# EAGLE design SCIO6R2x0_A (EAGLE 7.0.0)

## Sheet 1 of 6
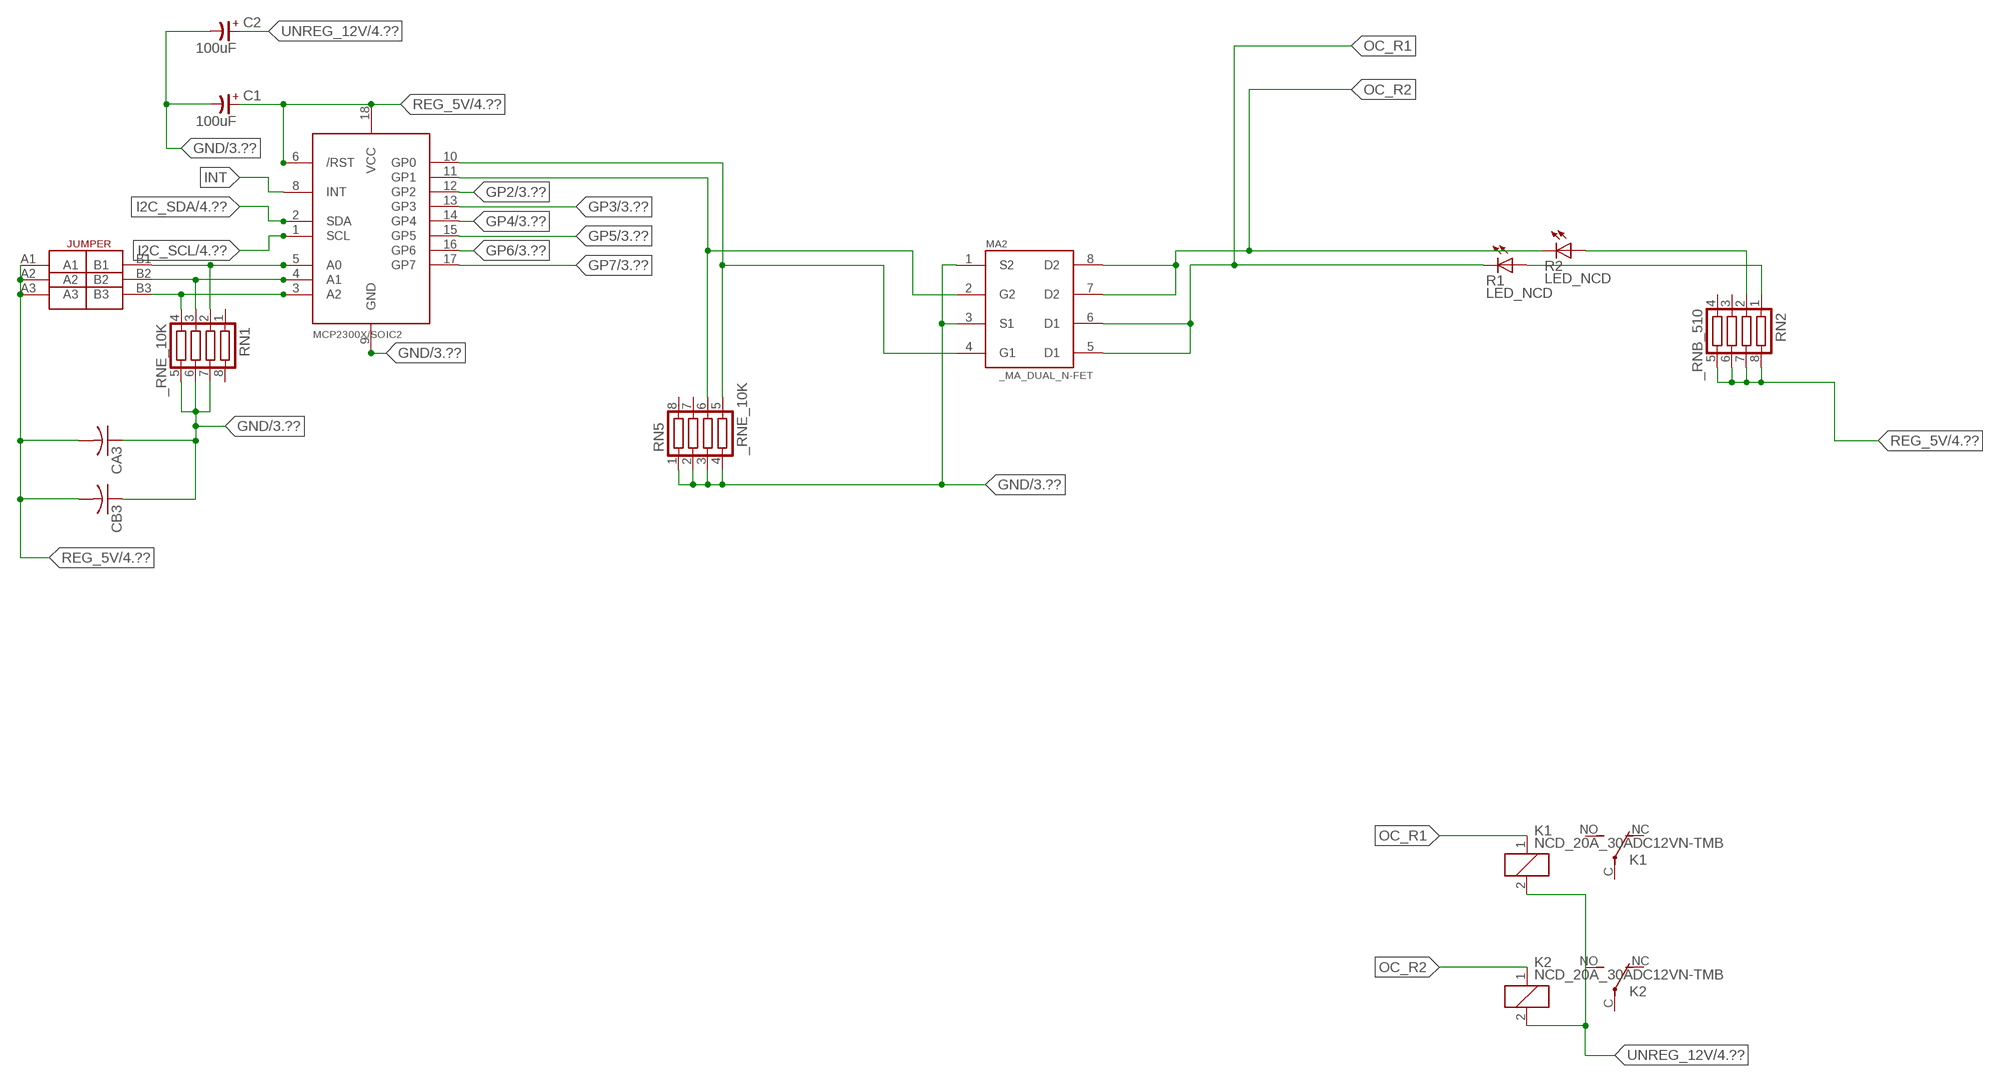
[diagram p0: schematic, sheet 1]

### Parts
C1  100uF  CP-E-025X060  [E-025X060]
C2  100uF  CP-E-025X060  [E-025X060]
CA3  CC1206KRX7R9BB104C1206K  [CC1206KRX7R9BB104]
CB3  TMK316F106ZL-TC1206K  [TMK316F106ZL-T]
IC2  MCP2300X/SO  [SO18W]
K1  NCD_20A_30ADC12VN-TMB  [JT-TMB]
K2  NCD_20A_30ADC12VN-TMB  [JT-TMB]
MA2  _MA_DUAL_N-FET  [_MA_DUAL_N-FET]
R1  LED_NCD  [CHIPLED_0603]
R2  LED_NCD  [CHIPLED_0603]
RN1  _RNE_10K  [RNE]
RN2  _RNB_510  [RNB]
RN5  _RNE_10K  [RNE]
U$18  JUMPER_3X2  [JUMPER_3X2]

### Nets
GND: C1.- C2.- CA3.1 CB3.1 IC2.9(GND) MA2.1(S2) MA2.3(S1) RN1.5 RN1.6 RN1.7 RN5.1 RN5.2 RN5.3 RN5.4 ; also sheet 3,4,6
GP2: IC2.12(GP2) ; also sheet 3
GP3: IC2.13(GP3) ; also sheet 3
GP4: IC2.14(GP4) ; also sheet 3
GP5: IC2.15(GP5) ; also sheet 3
GP6: IC2.16(GP6) ; also sheet 3
GP7: IC2.17(GP7) ; also sheet 3
I2C_SCL: IC2.1(SCL) ; also sheet 4
I2C_SDA: IC2.2(SDA) ; also sheet 4
INT: IC2.8(INT)
N$6: IC2.5(A0) RN1.2 U$18.B1
N$7: IC2.4(A1) RN1.3 U$18.B2
N$8: IC2.3(A2) RN1.4 U$18.B3
N$22: IC2.11(GP1) MA2.2(G2) RN5.6
N$23: IC2.10(GP0) MA2.4(G1) RN5.5
N$31: R2.A RN2.2
N$32: R1.A RN2.1
OC_R1: K1.1(C1) MA2.5(D1) MA2.6(D1) R1.C
OC_R2: K2.1(C1) MA2.7(D2) MA2.8(D2) R2.C
REG_5V: C1.+ CA3.2 CB3.2 IC2.6(/RST) IC2.18(VCC) RN2.5 RN2.6 RN2.7 RN2.8 U$18.A1 U$18.A2 U$18.A3 ; also sheet 4,6
UNREG_12V: C2.+ K1.2(C2) K2.2(C2) ; also sheet 4
Unconnected: K1.C(COM) K1.NC K1.NO K2.C(COM) K2.NC K2.NO RN1.1 RN1.8 RN2.3 RN2.4 RN5.7 RN5.8

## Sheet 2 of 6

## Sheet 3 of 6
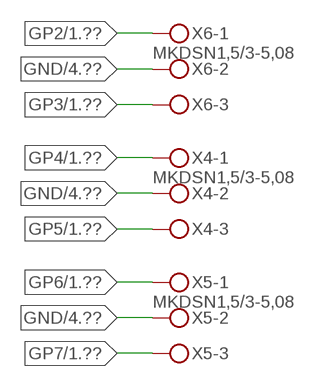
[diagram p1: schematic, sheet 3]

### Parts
X4  MKDSN1,5/3-5,08  [MKDSN1,5/3-5,08]
X5  MKDSN1,5/3-5,08  [MKDSN1,5/3-5,08]
X6  MKDSN1,5/3-5,08  [MKDSN1,5/3-5,08]

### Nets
GND: X4.2 X5.2 X6.2 ; also sheet 1,4,6
GP2: X6.1 ; also sheet 1
GP3: X6.3 ; also sheet 1
GP4: X4.1 ; also sheet 1
GP5: X4.3 ; also sheet 1
GP6: X5.1 ; also sheet 1
GP7: X5.3 ; also sheet 1

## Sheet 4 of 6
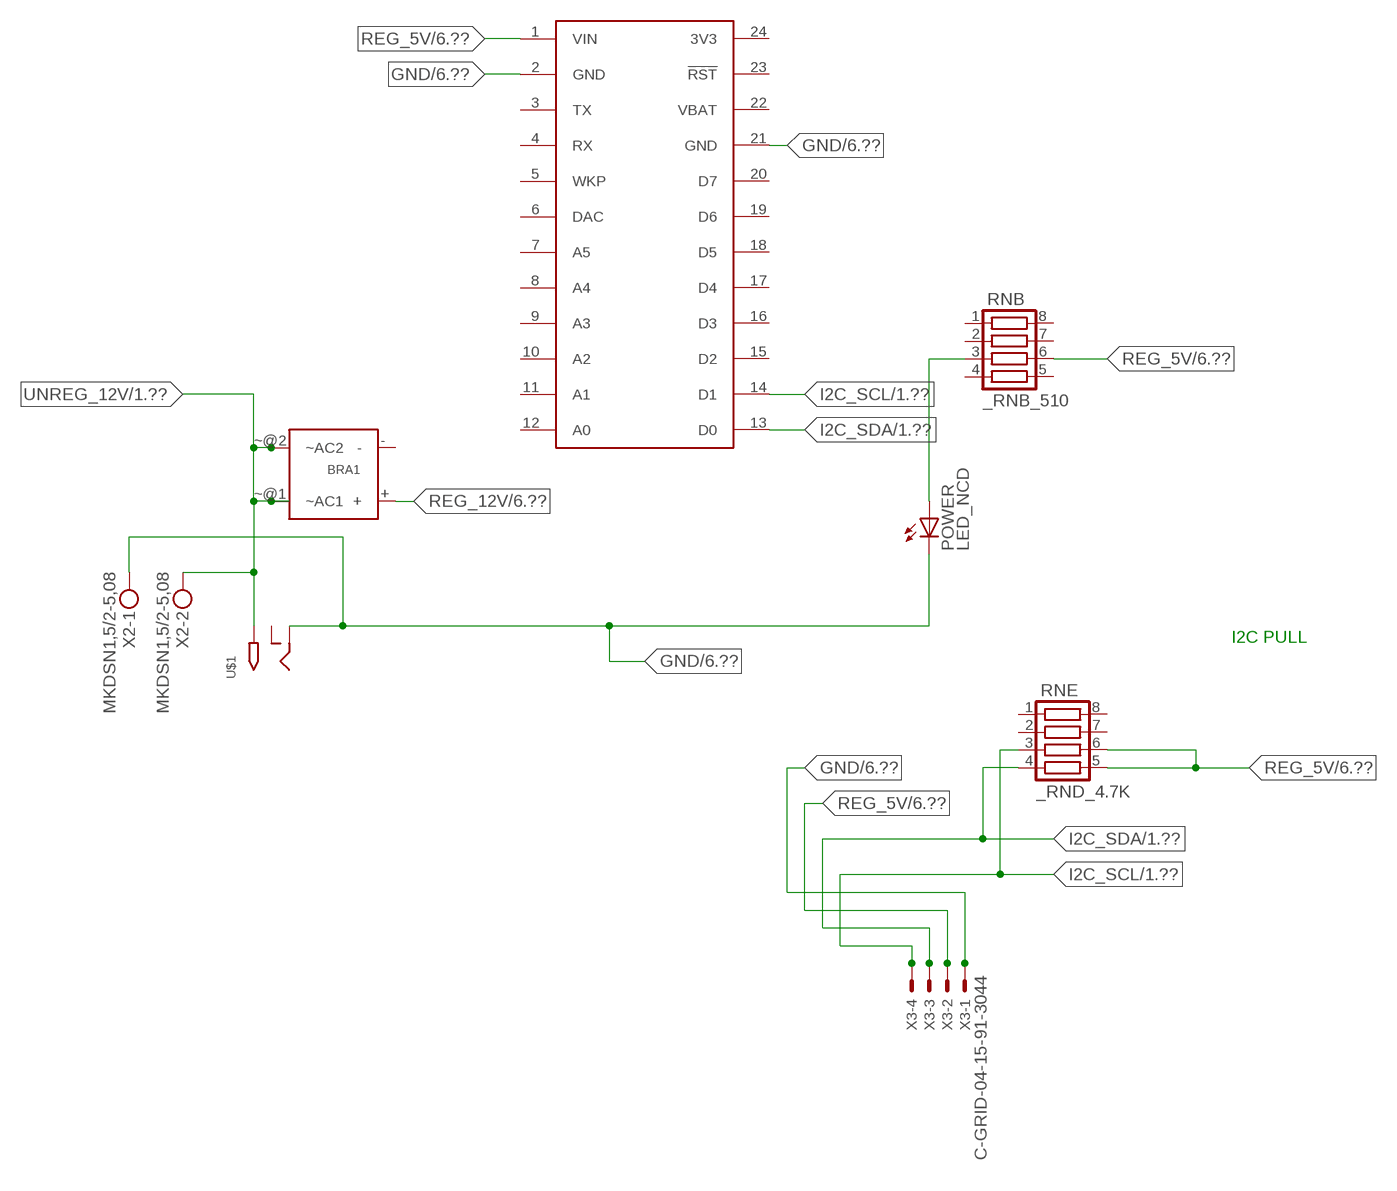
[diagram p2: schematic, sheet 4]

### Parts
BRA1  MB2S_  [MB2S]
POWER  LED_NCD  [CHIPLED_0603]
RNB  _RNB_510  [RNB]
RNE  _RND_4.7K  [RND]
S1  SPARK_CORECORE  [SPARK_CORE]
U$1  2.1MMJACK  [PJ-102A]
X2  MKDSN1,5/2-5,08  [MKDSN1,5/2-5,08]
X3  C-GRID-04-15-91-3044  [15-91-04]

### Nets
GND: POWER.C S1.2(GND) S1.21(GND) U$1.RING X2.1 X3.1 ; also sheet 1,3,6
I2C_SCL: RNE.3 S1.14(D1) X3.4 ; also sheet 1
I2C_SDA: RNE.4 S1.13(D0) X3.3 ; also sheet 1
N$2: POWER.A RNB.3
REG_5V: RNB.6 RNE.5 RNE.6 S1.1(VIN) X3.2 ; also sheet 1,6
REG_12V: BRA1.+ ; also sheet 6
UNREG_12V: BRA1.~@1(~AC1) BRA1.~@2(~AC2) U$1.TIP X2.2 ; also sheet 1
Unconnected: BRA1.- RNB.1 RNB.2 RNB.4 RNB.5 RNB.7 RNB.8 RNE.1 RNE.2 RNE.7 RNE.8 S1.3(TX) S1.4(RX) S1.5(WKP) S1.6(DAC) S1.7(A5) S1.8(A4) S1.9(A3) S1.10(A2) S1.11(A1) S1.12(A0) S1.15(D2) S1.16(D3) S1.17(D4) S1.18(D5) S1.19(D6) S1.20(D7) S1.23(!RST) U$1.RING_SW

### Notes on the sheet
- I2C PULL

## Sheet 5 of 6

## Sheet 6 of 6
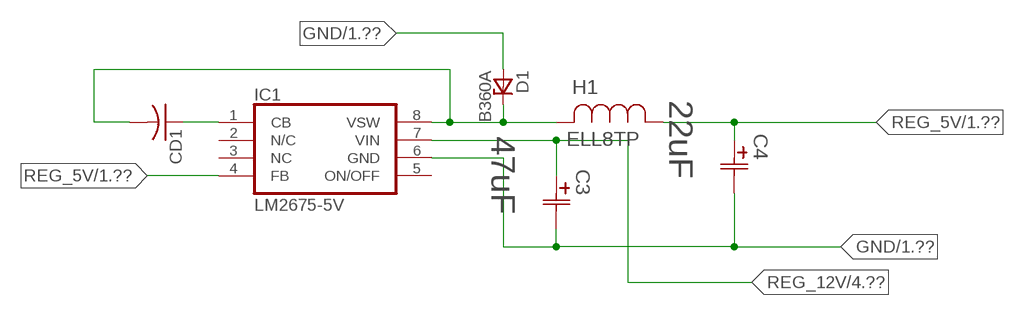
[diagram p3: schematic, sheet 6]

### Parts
C3  47uF  490-5463-6-NDCAP  [C2917(7343)-Y]
C4  22uF  490-5463-6-NDCAP  [C2917(7343)-Y]
CD1  _CD_10NF_50VC1206K  [_CD_10NF_50V]
D1  B360A  [DO214AC_ZENER]
H1  ELL8TP  [IND_ELL8TP]
IC1  LM2675-5V  LM2675  [SO-8]

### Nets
GND: C3.2(C2) C4.2(C2) D1.A IC1.6(GND) ; also sheet 1,3,4
N$1: CD1.2 D1.C H1.2 IC1.8(VSW)
N$3: CD1.1 IC1.1(CB)
REG_5V: C4.1(C1) H1.1 IC1.4(FB) ; also sheet 1,4
REG_12V: C3.1(C1) IC1.7(VIN) ; also sheet 4
Unconnected: IC1.2(N/C) IC1.5(ON/OFF)

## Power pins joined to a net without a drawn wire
3V3: S1.24(3V3)
NC: IC1.3(NC)
VBAT: S1.22(VBAT)

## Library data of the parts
BRA1 = NCD_ULTIMATE_LIBRARY:MB2S: Bridge Rectifier BRA MB2S 200V 500ma Digikey MB2S-TPMSTR-ND/MB2S-TP
C1 C2 = NCD_ULTIMATE_LIBRARY:CP-: Capacitors All Kinds POLARIZED CAP
C3 C4 = NCD_ULTIMATE_bhaskar:490-5463-6-ND: NCD CAP
CA3 = NCD_ULTIMATE_LIBRARY:CC1206KRX7R9BB104: Capacitor CA .1uF 50V SMT C1206K CC1206KRX7R9BB104
CB3 = NCD_ULTIMATE_LIBRARY:TMK316F106ZL-T: Capacitor CB 10uF SMT 1206 TMK316F106ZL-T
CD1 = NCD_ULTIMATE_LIBRARY:_CD_10NF_50V: Capacitor 10nF SMT
D1 = NCD_ULTIMATE_bhaskar:B360A: NCD DIODE B350A/B360A
H1 = NCD_ULTIMATE_bhaskar:ELL8TP: NCD coil
IC1 = NCD_ULTIMATE_bhaskar:LM2675: LM2675 NCD http://www.ti.com/lit/ds/symlink/lm2675.pdf
IC2 = NCD_ULTIMATE_LIBRARY:MCP2300X: Semiconductor Port Expander I/O 8-Bit I2C MCP23008 Inexpensive i2c i/o expander - 8 general purpose i/o pins with optional pullups
K1 K2 = NCD_ULTIMATE_LIBRARY:NCD_20A_30A: RELAY COMPACT ECONOMICAL 30 AMP. RELAY NAiS Source: http://www.mew-europe.com/.. en_ds_61212_0000.pdf
MA2 = NCD_ULTIMATE_LIBRARY:_MA_DUAL_N-FET: FET Dual N-Channel 8-SOIC NMOSFET Digikey 785-1064-2-ND/AO4842
POWER = NCD_ULTIMATE_bhaskar:LED_NCD
R1 R2 = NCD_ULTIMATE_LIBRARY:LED_NCD: LED Digikey 754-1132-2-ND/APT2012SRCPRV
RN1 RN5 = NCD_ULTIMATE_LIBRARY:_RNE_10K: Resistor Array RNE SMT 10K x 4 Single Resistor Source: http://www.ctscorp.com/components/Datasheets/CTSChipArrayDs.pdf Digikey 742C083103JPTR-ND/742C083103JP; OC_FARNELL: unknown; OC_NEWARK: unknown
RN2 RNB = NCD_ULTIMATE_LIBRARY:_RNB_510: Resistor Array RNB SMT 510 x 4 Single Resistor Source: http://www.ctscorp.com/components/Datasheets/CTSChipArrayDs.pdf Digikey 742C083511JPTR-ND/ 742C083511JP; OC_FARNELL: unknown; OC_NEWARK: unknown
RNE = NCD_ULTIMATE_LIBRARY:_RND_4.7K: Resistor Array RND SMT 4.7K x 4 Single Resistor Source: http://www.ctscorp.com/components/Datasheets/CTSChipArrayDs.pdf Digikey 742C083472JPTR-ND/742C083472JP; OC_FARNELL: unknown; OC_NEWARK: unknown
S1 = Spark:SPARK_CORE
U$1 = NCD_ULTIMATE_CONNECTORS:2.1MMJACK: 2.1mm x 5.5mm DC jack with internal switch. Digikey part #PJ-102A, 4UCON part #05537 By microbuilder.eu
U$18 = NCD_ULTIMATE_CONNECTORS:JUMPER_3X2
X2 = NCD_ULTIMATE_CONNECTORS:MKDSN1,5/2-5,08: MKDSN 1,5/ 2-5,08 Printklemme
X3 = NCD_ULTIMATE_CONNECTORS:C-GRID-04: CONNECTOR 4-Pos I2C wire to board 2.54 mm (0.100") pitch header Digikey WM1342-ND/0015912045; OC_FARNELL: unknown; OC_NEWARK: unknown
X4-X6 = NCD_ULTIMATE_CONNECTORS:MKDSN1,5/3-5,08: MKDSN 1,5/ 3-5,08 Printklemme Nennstrom: 13,5 A Nennspannung: 250 V Rastermaß: 5,08 mm Polzahl: 3 Anschlussart: Schraubanschluss Montage: Löten Anschlussrichtung Leiter/Platine: 0 ° Artikelnummer: 1729131 Source: http://eshop.phoenixcontact.com .. 1729131.pdf

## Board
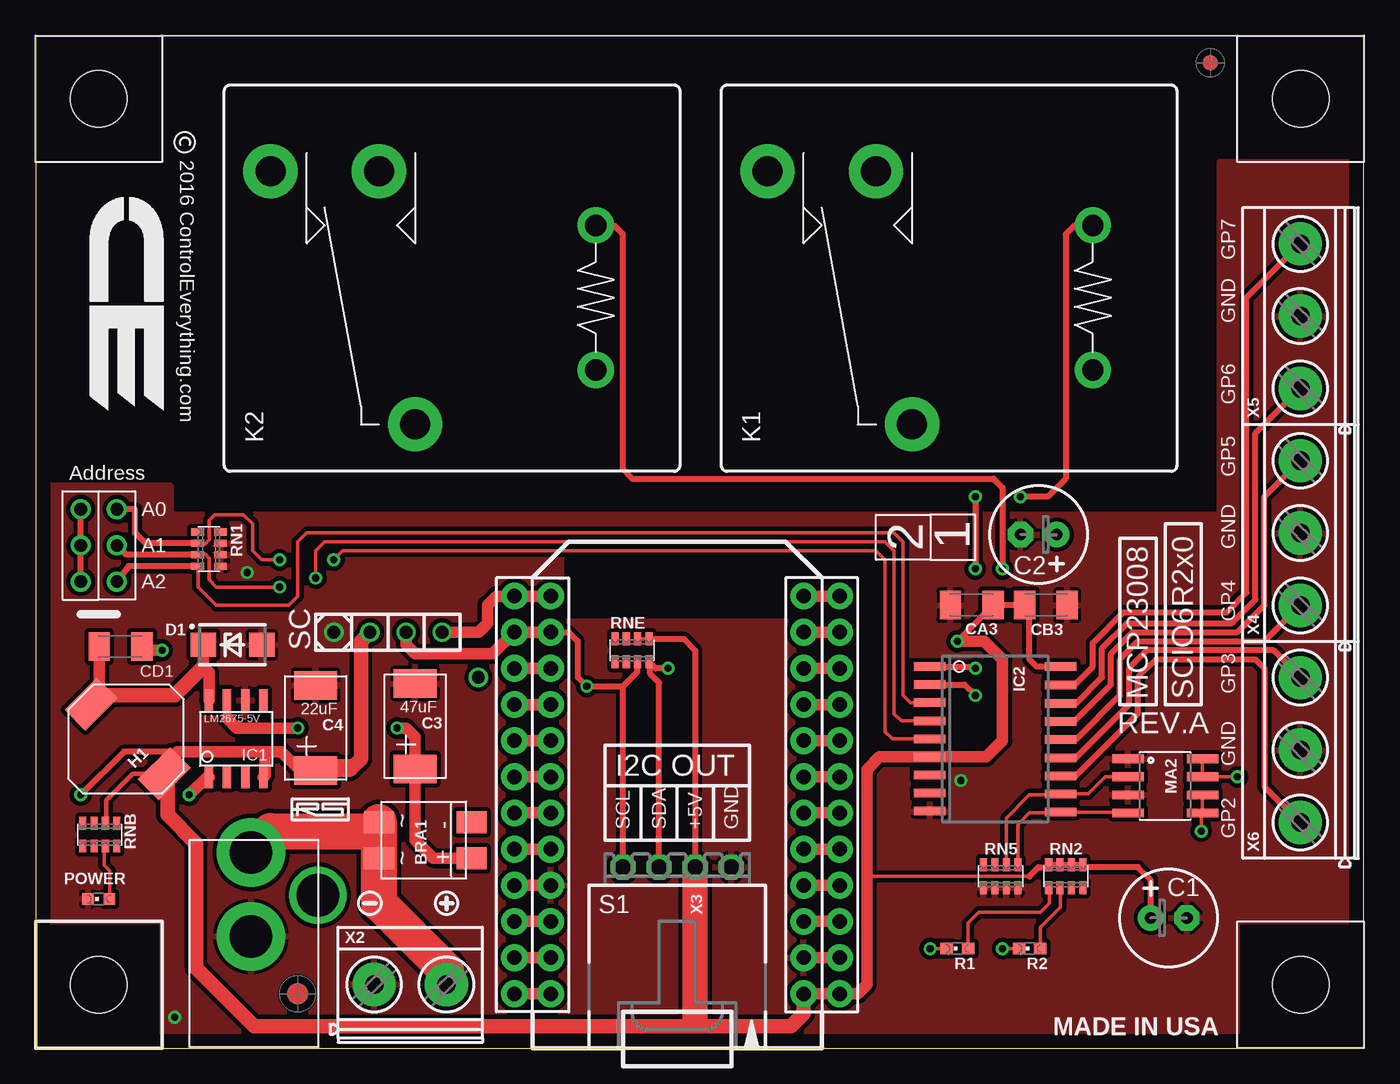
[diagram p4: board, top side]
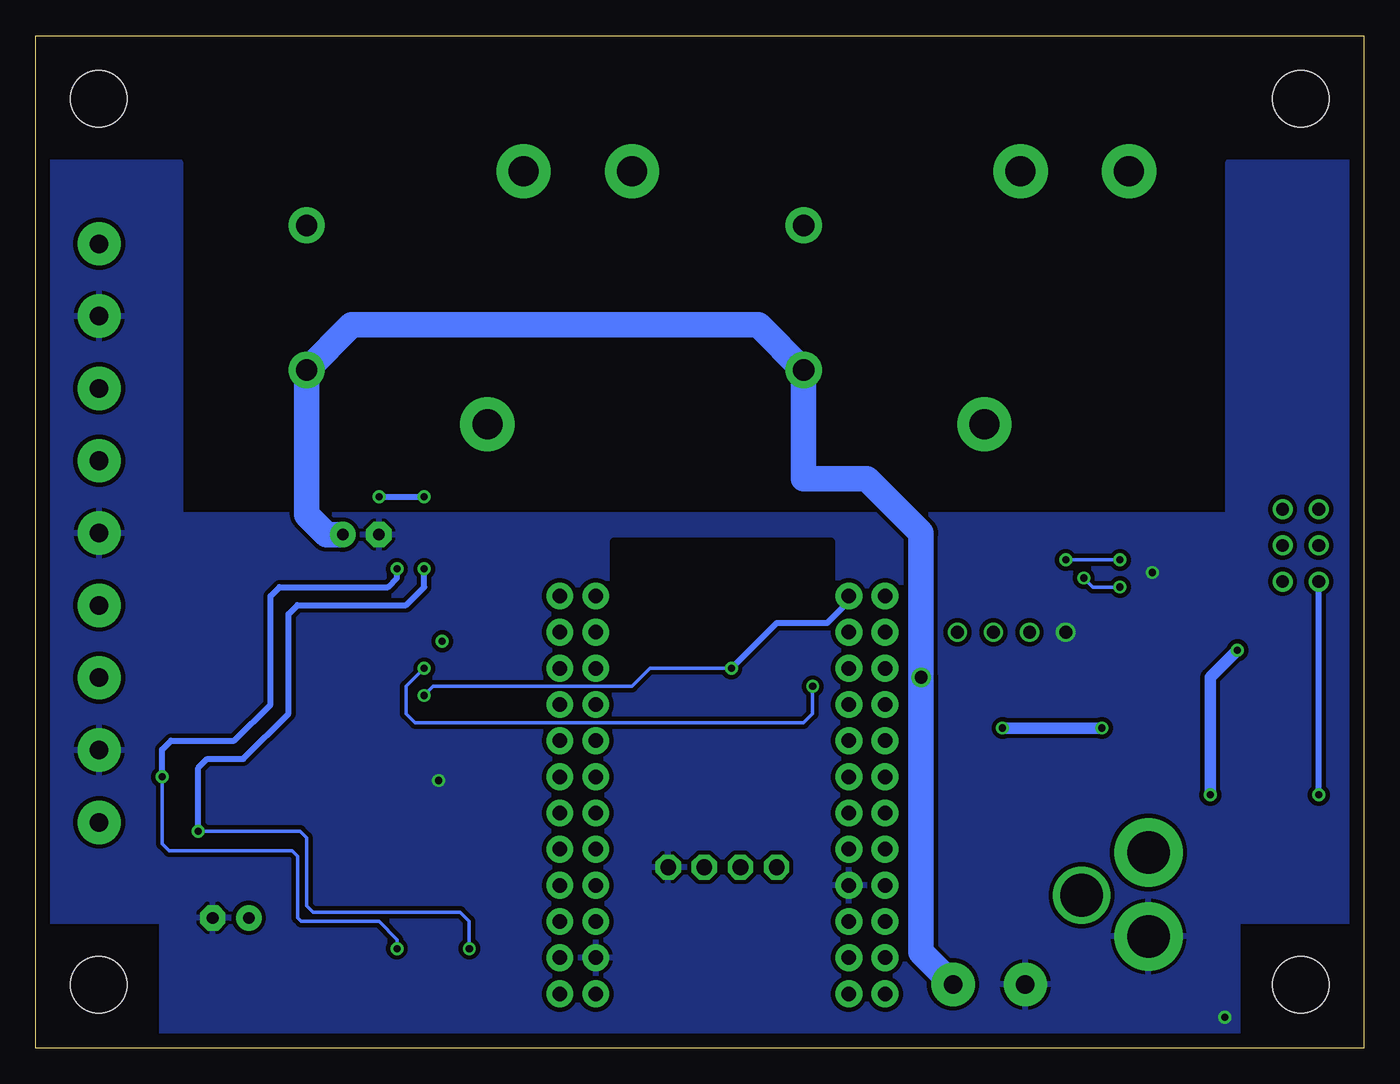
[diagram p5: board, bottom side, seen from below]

Size 93.34 x 71.12 mm. Coordinates in mm from the lower left corner, seen from the top.
Outline: 0,59.99 0,59.05
Outline: 0,59.05 0,0 75.56,0 93.34,0 93.34,71.12 0,71.12 0,59.05
Copper layers (1*16): Top 0.035mm / dielectric 1.5mm / Bottom 0.035mm
Design rules "default": minimum track width 10mil, minimum drill 24mil, track to track 8mil, track to pad 8mil, pad to pad 8mil, via to via 8mil, smd to smd 8mil, copper to edge 40mil, drill to drill 8mil, minimum pad ring 10mil, minimum via ring 8mil, stop-mask expansion 4mil, vias tented up to drill 0mil, thermal gap 10mil
Holes 3.96 mm at 4.45,4.45 4.45,4.45

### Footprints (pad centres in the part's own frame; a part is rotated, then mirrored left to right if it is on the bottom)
MB2S = smd 1.55 x 2.1: + 0,-6.5; - 2.54,-6.5; ~@1 0,0; ~@2 2.54,0
E-025X060 = drill 0.813 pad 1.778: + -1.27,0 | drill 0.813 pad 1.778 octagon: - 1.27,0
C2917(7343)-Y = smd 2 x 3: 1 -3,0; 2 3,0
CC1206KRX7R9BB104 = smd 1.5 x 2: 1 -1.5,0; 2 1.5,0
TMK316F106ZL-T = smd 1.5 x 2: 1 -1.5,0; 2 1.5,0
_CD_10NF_50V = smd 1.5 x 2: 1 -1.5,0; 2 1.5,0
DO214AC_ZENER = smd 1.8 x 1.7: A 2.05,0; C -2.05,0
IND_ELL8TP = smd 2.054 x 3.2 rotated 45: 1 -2.442,-2.696; 2 2.442,2.442
SO-8 = smd 0.6 x 1.55: 1 -1.905,-2.69; 2 -0.635,-2.69; 3 0.635,-2.69; 4 1.905,-2.69; 5 1.905,2.71; 6 0.635,2.71; 7 -0.635,2.71; 8 -1.905,2.71
SO18W = smd 0.6 x 2.2: 1 -4.445,-4.6; 2 -3.175,-4.6; 3 -1.905,-4.6; 4 -0.635,-4.6; 5 0.635,-4.6; 6 1.905,-4.6; 7 3.175,-4.6; 8 4.445,-4.6; 9 5.715,-4.6; 10 5.775,4.6; 11 4.505,4.6; 12 3.235,4.6; 13 1.965,4.6; 14 0.695,4.6; 15 -0.575,4.6; 16 -1.845,4.6; 17 -3.145,4.6; 18 -4.445,4.6
JT-TMB = drill 1.5 pad 2.54: 1 5.08,0; 2 -5.08,0 | drill 2.1 pad 3.81: C -8.89,12.7; NC 8.89,22.86; NO 8.89,15.24
_MA_DUAL_N-FET = smd 0.61 x 2.21: 1 -1.905,-2.616; 2 -0.635,-2.616; 3 0.635,-2.616; 4 1.905,-2.616; 5 1.905,2.616; 6 0.635,2.616; 7 -0.635,2.616; 8 -1.905,2.616
CHIPLED_0603 = smd 0.8 x 0.8: A 0,-0.75; C 0,0.75
CHIPLED_0603' = smd 0.8 x 0.876: A 0,-0.75; C 0,0.75
RNE = smd 0.5 x 0.9: 1 -1.2,-0.8; 2 -0.4,-0.8; 3 0.4,-0.8; 4 1.2,-0.8; 5 1.2,0.8; 6 0.4,0.8; 7 -0.4,0.8; 8 -1.2,0.8
RNB = smd 0.5 x 0.9: 1 -1.2,-0.8; 2 -0.4,-0.8; 3 0.4,-0.8; 4 1.2,-0.8; 5 1.2,0.8; 6 0.4,0.8; 7 -0.4,0.8; 8 -1.2,0.8
RND = smd 0.5 x 0.9: 1 -1.2,-0.8; 2 -0.4,-0.8; 3 0.4,-0.8; 4 1.2,-0.8; 5 1.2,0.8; 6 0.4,0.8; 7 -0.4,0.8; 8 -1.2,0.8
SPARK_CORE = drill 1.016 pad 1.88: 1 -8.89,13.97; 2 -8.89,11.43; 3 -8.89,8.89; 4 -8.89,6.35; 5 -8.89,3.81; 6 -8.89,1.27; 7 -8.89,-1.27; 8 -8.89,-3.81; 9 -8.89,-6.35; 10 -8.89,-8.89; 11 -8.89,-11.43; 12 -8.89,-13.97; 13 8.89,-13.97; 14 8.89,-11.43; 15 8.89,-8.89; 16 8.89,-6.35; 17 8.89,-3.81; 18 8.89,-1.27; 19 8.89,1.27; 20 8.89,3.81; 21 8.89,6.35; 22 8.89,8.89; 23 8.89,11.43; 24 8.89,13.97; 25 -11.43,13.97; 26 -11.43,11.43; 27 -11.43,8.89; 28 -11.43,6.35; 29 -11.43,3.81; 30 -11.43,1.27; 31 -11.43,-1.27; 32 -11.43,-3.81; 33 -11.43,-6.35; 34 -11.43,-8.89; 35 -11.43,-11.43; 36 -11.43,-13.97; 37 11.43,13.97; 38 11.43,11.43; 39 11.43,8.89; 40 11.43,6.35; 41 11.43,3.81; 42 11.43,1.27; 43 11.43,-1.27; 44 11.43,-3.81; 45 11.43,-6.35; 46 11.43,-8.89; 47 11.43,-11.43; 48 11.43,-13.97
PJ-102A = drill 3 pad 4.8: RING 0.1,-3.39; TIP 0.1,-9.29 | drill 3 pad 3.251: RING_SW -4.6,-6.29
PCB_MOUNTING_HOLE = hole 3.962: 4.445,4.445
JUMPER_3X2 = drill 0.9: A1 0,5.08; A2 0,2.54; A3 0,0; B1 2.54,5.08; B2 2.54,2.54; B3 2.54,0
MKDSN1,5/2-5,08 = drill 1.3 pad 3.048: 1 -2.561,0.025; 2 2.519,0.025
15-91-04 = drill 1.1 pad 1.778 octagon: 1 -3.81,-7.62; 2 -1.27,-7.62; 3 1.27,-7.62; 4 3.81,-7.62
MKDSN1,5/3-5,08 = drill 1.3 pad 3.048: 1 -7.641,0.025; 2 -2.561,0.025; 3 2.519,0.025

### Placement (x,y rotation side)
BRA1  24.13,13.34 90 top
C1  79.63,9.14 0 top
C2  70.48,36.07 180 top
C3  26.67,22.61 90 top
C4  19.68,22.48 90 top
CA3  65.79,31.12 0 top
CB3  70.99,31.12 180 top
CD1  5.97,28.19 180 top
D1  13.84,28.32 0 top
H1  6.35,21.72 90 top
IC1  14.1,21.72 0 top
IC2  67.44,22.35 270 top
K1  74.3,52.7 90 top
K2  39.37,52.7 90 top
MA2  79.38,18.41 270 top
POWER  4.45,10.48 90 top
R1  LED_NCD  [CHIPLED_0603']  64.77,6.98 90 top
R2  LED_NCD  [CHIPLED_0603']  69.85,6.98 90 top
RN1  12.19,35.05 270 top
RN2  72.39,12.07 0 top
RN5  67.82,12.07 0 top
RNB  4.51,14.99 0 top
RNE  41.91,27.94 0 top
S1  45.09,17.78 180 top
U$1  15.24,4.45 180 top
U$4  PCB_MOUNTING_HOLE  [PCB_MOUNTING_HOLE]  93.34,62.23 90 top
U$6  PCB_MOUNTING_HOLE  [PCB_MOUNTING_HOLE]  93.34,0 90 top
U$10  [VISION_REF15]  18.41,3.81 0 top
U$11  PCB_MOUNTING_HOLE  [PCB_MOUNTING_HOLE]  8.89,62.23 90 top
U$18  3.17,32.77 0 top
U$19  [VISION_REF10]  82.55,69.22 0 top
U$21  [ICON_USA]  71.5,0.89 0 top
U$22  [ICON_MINUS]  23.5,10.16 180 top
U$24  [ICON_PLUS]  28.89,10.16 90 top
X2  26.35,4.45 0 top
X3  45.09,5.08 180 top
X4  88.9,38.73 90 top
X5  88.9,53.97 90 top
X6  88.9,23.5 90 top

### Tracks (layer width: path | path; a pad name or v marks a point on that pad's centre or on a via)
GND  (via drill 0.5, 0.9)
  other vias: 14.86,33.4 65.02,18.8 9.78,2.16 20.95,29.21
  pour Bottom (isolate 0.305): -1.91,8.89 8.89,8.89 8.89,0 84.45,0 84.45,8.89 92.71,8.89 92.71,62.23 83.19,62.23 83.19,37.46 9.53,37.46 9.53,62.23 -1.91,62.23
  pour Top (isolate 0.305): -3.81,8.89 8.89,8.89 8.89,0 84.45,0 84.45,8.89 92.71,8.89 92.71,62.23 83.19,62.23 83.19,37.46 9.53,37.46 9.53,39.5 -3.81,39.5
GP2
  Top 0.406: IC2.12 73.09,19.12 77.47,23.5 77.47,26.04 78.74,27.3 85.72,27.3 86.36,26.67 86.36,18.37 X6.1
GP3
  Top 0.406: X6.3 88.88,26.06 87,27.94 78.11,27.94 76.83,26.67 76.83,24.13 73.03,20.32 72.1,20.32 IC2.13
GP4
  Top 0.406: IC2.14 73.09,21.66 76.2,24.77 76.2,27.3 77.47,28.57 86.36,28.57 X4.1
GP5
  Top 0.406: IC2.15 72.97,22.93 75.56,25.53 75.56,27.69 77.09,29.21 84.45,29.21 86.36,31.12 86.36,38.74 X4.3
GP6
  Top 0.406: IC2.16 73.09,24.2 74.93,26.04 74.93,28.07 76.71,29.85 84.07,29.85 85.72,31.5 85.72,43.18 X5.1
GP7
  Top 0.406: IC2.17 73,25.5 74.3,26.8 74.3,28.45 76.45,30.61 83.69,30.61 85.09,32 85.09,52.71 X5.3
I2C_SCL  (via drill 0.5, 0.9)
  Top 0.406: IC2.1 65.91,26.8 v66.04,26.67 | X3.4 41.27,25.4 | 41.27,25.4 42.29,26.42 42.29,27.12 RNE.3 | S1.14 37.47,29.21 38.1,28.57 38.1,26.04 v38.73,25.4 41.27,25.4
  Top 0.813: v26.04,29.21 26.04,28.32 26.67,27.69 32.13,27.69 33.66,29.21
  Bottom 0.254: v38.73,25.4 38.73,23.5 39.37,22.86 66.67,22.86 67.31,23.5 67.31,25.4 v66.04,26.67
I2C_SDA  (via drill 0.5, 0.9)
  Top 0.406: IC2.2 65.28,25.53 v66.04,24.77 | X3.3 43.81,25.65 43.18,26.29 43.18,27.07 RNE.4 43.58,26.67 v44.45,26.67
  Top 0.813: v28.57,29.21 31.11,29.21 31.75,29.85 31.75,31.12 32.38,31.75 33.66,31.75
  Bottom 0.254: v44.45,26.67 50.16,26.67 51.44,25.4 65.41,25.4 v66.04,24.77
  Bottom 0.406: S1.13 36.2,31.37 37.72,29.85 41.27,29.85 v44.45,26.67
N$1
  Top 0.813: H1.2 3.88,24.77 | D1.C 11.79,26.78 12.19,26.38 IC1.8 | CD1.2 4.47,24.79 4.45,24.77
  Top 1.016: 3.88,24.77 4.45,24.77 9.78,24.77 11.79,26.78
N$2
  Top 0.254: POWER.A 5.2,12.46 4.83,12.83 4.83,14.1 RNB.3
  Top 0.406: 4.95,14.14 RNB.3
N$3  (via drill 0.5)
  Top 0.813: IC1.1 12.04,19.03 v10.79,17.78 | v8.89,27.94 7.72,27.94 CD1.1
  Bottom 0.813: v10.79,17.78 10.79,26.04 v8.89,27.94
N$6  (via drill 0.5)
  Top 0.254: IC2.5 60.2,21.72 59.69,22.23 59.69,34.29 59.05,34.92 21.59,34.92 v20.95,34.29 | v17.14,34.29 15.88,34.29 15.24,34.92 15.24,36.83 14.61,37.46 12.57,37.46 12.19,37.08 12.19,35.69 11.94,35.43 11.41,35.43 RN1.2
  Top 0.406: RN1.2 7.73,35.45 6.99,36.2 6.99,37.85 U$18.B1
  Bottom 0.254: v20.95,34.29 v17.14,34.29
N$7  (via drill 0.5)
  Top 0.254: IC2.4 60.83,22.99 60.33,23.5 60.33,34.92 59.69,35.56 20.32,35.56 19.68,34.92 v19.68,33.02 | v17.14,32.38 12.7,32.38 12.19,32.89 12.19,34.42 11.94,34.67 11.41,34.67 RN1.3
  Top 0.406: RN1.3 6.37,34.65 U$18.B2
  Bottom 0.254: v19.68,33.02 19.05,32.38 v17.14,32.38
N$8
  Top 0.254: IC2.3 61.47,24.26 60.96,24.77 60.96,35.56 60.33,36.2 19.05,36.2 18.41,35.56 18.41,31.75 17.78,31.12 12.7,31.12 11.43,32.38 11.43,33.81 RN1.4
  Top 0.406: RN1.4 6.53,33.85 U$18.B3
N$22
  Top 0.254: MA2.2 75.18,19.05 73.98,17.85 IC2.11 71.97,17.78 69.85,17.78 68.22,16.15 RN5.6
N$23
  Top 0.254: MA2.4 76.69,16.58 IC2.10 71.97,16.51 69.85,16.51 69.02,15.68 RN5.5
N$31
  Top 0.254: R2.A 70.6,8.5 72.01,9.91 72.01,11.25 RN2.2
N$32
  Top 0.254: R1.A 65.52,8.75 66.29,9.52 70.61,9.52 71.25,10.16 71.25,11.21 RN2.1
OC_R1  (via drill 0.5)
  Top 0.254: R1.C v62.87,6.98 | v81.92,15.24 81.92,16.43 MA2.5 MA2.6
  Top 0.406: K1.1 73.03,57.78 72.39,57.15 72.39,40 71.12,38.73 v69.22,38.73 | v66.04,38.73 v66.04,33.66
  Bottom 0.254: v62.87,6.98 62.87,8.89 63.5,9.52 73.84,9.52 74.3,9.98 74.3,14.78 74.75,15.24 v81.92,15.24
  Bottom 0.406: v81.92,15.24 81.92,19.69 81.28,20.32 78.74,20.32 75.56,23.5 75.56,30.48 74.93,31.12 67.31,31.12 66.04,32.38 v66.04,33.66 | v69.22,38.73 v66.04,38.73
OC_R2  (via drill 0.5)
  Top 0.254: R2.C v67.94,6.98 | v84.45,19.05 MA2.7 MA2.8
  Top 0.406: v67.94,33.66 67.94,39.37 67.31,40 41.91,40 41.27,40.64 41.27,57.15 40.64,57.78 K2.1
  Bottom 0.254: v67.94,6.98 67.94,7.62 69.22,8.89 74.68,8.89 74.93,9.14 74.93,13.46 75.31,13.84 83.95,13.84 84.45,14.35 v84.45,19.05
  Bottom 0.406: v84.45,19.05 84.45,20.96 83.82,21.59 79.38,21.59 76.83,24.13 76.83,31.75 76.2,32.38 68.58,32.38 67.94,33.02 v67.94,33.66
REG_5V  (via drill 0.5, 0.9)
  Top 0.229: 58.42,12.07 69.85,12.07
  Top 0.254: RNE.6 RNE.5
  Top 0.305: H1.1 6.83,19.28 4.95,17.4 4.95,15.83 RNB.6
  Top 0.406: U$18.A3 U$18.A2 U$18.A1 | IC2.18 70.36,26.8 69.85,27.3 69.85,30.76 CB3.2 CA3.2 65.38,29.19 v64.77,28.57 | 62.71,20.32 IC2.6 | 69.85,12.07 70.48,12.7 71.03,12.7 RN2.8 RN2.7 RN2.6 RN2.5 73.75,12.7 77.47,12.7 78.36,11.81 C1.+ | RNE.5 45.55,28.74 46.35,27.94 X3.2 | 9.96,20.83 6.22,20.83 v3.17,17.78
  Top 0.61: 69.22,31.75 69.22,31.39 CB3.2
  Top 0.813: 16.13,20.83 9.96,20.83 H1.1 | 16.13,20.83 17.27,20.83 18.41,19.69 20.75,19.69 C4.1 | IC1.4 16.13,19.15 16.13,20.83 | 56.52,3.81 57.78,3.81 58.42,4.45 58.42,12.07 58.42,19.56 59.31,20.45 IC2.6 66.8,20.45 67.94,21.59 67.94,27.3 66.67,28.57 v64.77,28.57
  Top 1.016: 46.35,2.16 46.35,1.52 | 46.35,1.52 15.37,1.52 11.3,5.59 11.3,14.35 9.27,16.38 9.27,18.41 H1.1 | 22.05,19.69 22.23,19.69 22.86,20.32 22.86,28.57 v23.5,29.21 | S1.1 53.98,2.41 53.09,1.52 46.35,1.52
  Top 1.27: 20.75,19.69 22.05,19.69
  Top 1.778: X3.2 46.35,2.16
  Bottom 0.406: v3.17,17.78 U$18.A3
REG_12V  (via drill 0.5)
  Top 0.61: IC1.7 13.46,23.16 | 14.1,22.48 14.15,22.48
  Top 0.813: v18.41,22.48 14.15,22.48 13.46,23.16 | v25.4,22.48 26.04,22.48 26.67,21.84 C3.1 26.67,14.61 27.94,13.34 BRA1.+
  Bottom 0.813: v18.41,22.48 v25.4,22.48
UNREG_12V  (via drill 0.9)
  Top 2.54: X2.2 28.87,5.42 24.13,10.16 BRA1.~@1 24.13,15.24 | 24.13,15.24 BRA1.~@2 | U$1.TIP 15.14,13.87 16.51,15.24 24.13,15.24
  Bottom 1.778: X2.2 31.11,6.71 v31.11,26.04 31.11,36.2 34.92,40 39.37,40 K2.2 42.55,50.8 71.12,50.8 K1.2 74.3,37.46 72.9,36.07 C2.+

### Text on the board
tNames: 2016 ControlEverything.com | GP7 | GND | GP6 | Address | GP5 | A0 | A1 | 2 | 1 | GND | A2 | GP4 | SC | GP3 | MCP23008 | SCIO6R2x0 | REV.A | GND | I2C OUT | SCL | SDA | +5V | GND | GP2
